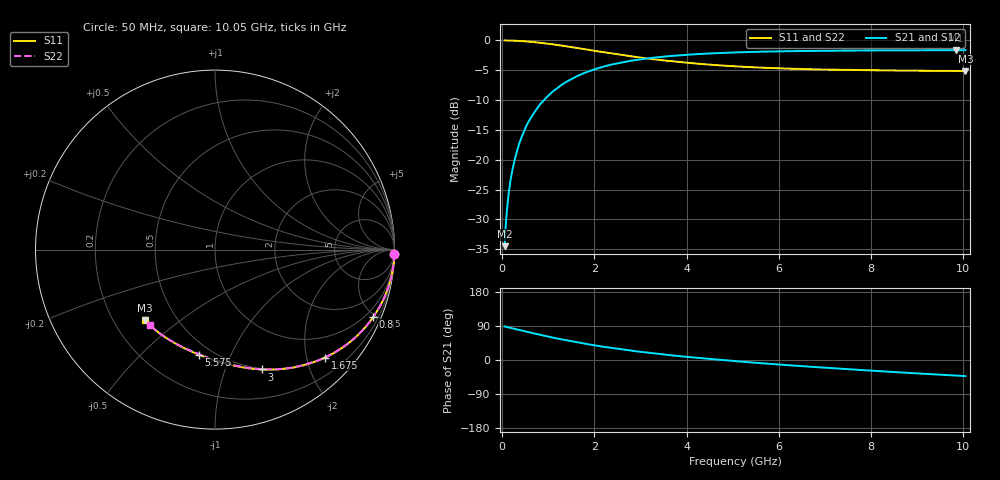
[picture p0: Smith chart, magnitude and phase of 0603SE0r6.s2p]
! AVX Thin Film Operation		Date: August 2001
! Description: Accu-P® Series, Thin Film, SMD, RF Capacitor
! Part Number: 06035J0R6ABT
! 50 MHz  -  10.05 GHz
! Serial Measurements
# mhz S db R 50
!	S11		S21		S12		S22
!	dB	Phase	dB	Phase	dB	Phase	dB	Phase
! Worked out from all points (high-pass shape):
!   401 points, 50 MHz to 10.05 GHz, reference 50 ohm
!   highest |S21| = -1.63 dB at 9.85 GHz (marker M1); lowest = -34.5 dB at 50 MHz (marker M2)
!   |S21| within 3 dB of the highest: 2.09 GHz to end of sweep
!   lowest |S11| = -5.1 dB at 10.05 GHz (marker M3), VSWR 3.49, Z = 16.6 - j18.9 ohm
!   |S11| at or under -10 dB: nowhere
!   |S22| runs from -5.1 to 0.0 dB; largest |S21 - S12| = 0
!   S11 on the Smith chart (normalised r, x): 50 MHz: 1, -77; 800 MHz: 0.53, -4.85; 1.675 GHz: 0.51, -2.35; 3 GHz: 0.49, -1.35; 5.575 GHz: 0.42, -0.77; 10.05 GHz: 0.33, -0.38
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50  -0.00 -1.5  -34.50 88.5  -34.50 88.5  -0.00 -1.5
75  -0.00 -2.2  -31.00 87.8  -31.00 87.8  -0.00 -2.2
125  -0.01 -3.7  -26.57 86.3  -26.57 86.3  -0.01 -3.7
175  -0.02 -5.2  -23.64 84.8  -23.64 84.8  -0.02 -5.2
225  -0.03 -6.7  -21.52 83.3  -21.52 83.3  -0.03 -6.7
300  -0.06 -8.9  -19.08 81.1  -19.08 81.1  -0.06 -8.9
400  -0.10 -11.8  -16.60 78.2  -16.60 78.2  -0.10 -11.8
525  -0.17 -15.4  -14.30 74.6  -14.30 74.6  -0.17 -15.4
800  -0.37 -23.0  -10.93 67.0  -10.93 67.0  -0.37 -23.0
1200  -0.77 -33.5  -7.92 56.5  -7.92 56.5  -0.77 -33.5
1675  -1.32 -44.5  -5.81 45.5  -5.81 45.5  -1.32 -44.4
1725  -1.39 -45.6  -5.63 44.4  -5.63 44.4  -1.39 -45.5
2300  -2.10 -57.0  -4.18 33.0  -4.18 33.0  -2.10 -56.8
3000  -2.88 -68.5  -3.17 21.6  -3.17 21.6  -2.87 -68.2
3400  -3.26 -74.2  -2.79 15.9  -2.79 15.9  -3.26 -73.7
4175  -3.86 -84.0  -2.32 6.3  -2.32 6.3  -3.85 -83.2
5050  -4.34 -93.4  -2.02 -3.0  -2.02 -3.0  -4.33 -92.4
5575  -4.55 -98.5  -1.90 -8.1  -1.90 -8.1  -4.54 -97.3
6725  -4.84 -109.3  -1.75 -18.1  -1.75 -18.1  -4.83 -107.3
8400  -5.03 -122.2  -1.66 -31.0  -1.66 -31.0  -5.01 -119.2
9850  -5.12 -133.2  -1.63 -41.2  -1.63 -41.2  -5.09 -129.2
10050  -5.13 -134.7  -1.63 -42.5  -1.63 -42.5  -5.11 -130.7
